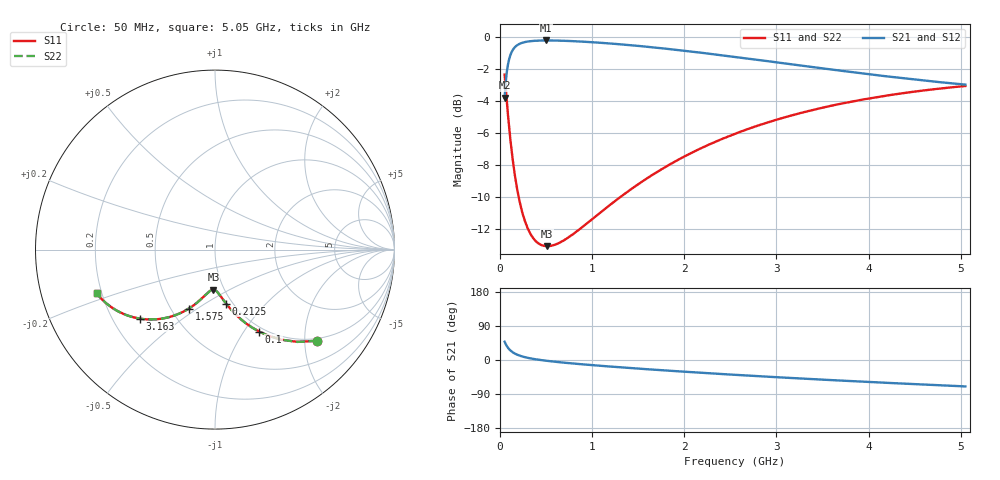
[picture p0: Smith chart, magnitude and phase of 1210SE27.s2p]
! AVX Thin Film Operation		Date: August 2001
! Description: Accu-P® Series, Thin Film, SMD, RF Capacitor
! Part Number: 12101J270FBT
! 50 MHz  -  5.05 GHz
! Serial Measurements
# mhz S db R 50
!	S11		S21		S12		S22
!	dB	Phase	dB	Phase	dB	Phase	dB	Phase
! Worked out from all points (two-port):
!   401 points, 50 MHz to 5.05 GHz, reference 50 ohm
!   highest |S21| = -0.22 dB at 500 MHz (marker M1); lowest = -3.8 dB at 50 MHz (marker M2)
!   |S21| within 3 dB of the highest: 57.29 MHz to end of sweep
!   lowest |S11| = -13.0 dB at 512.5 MHz (marker M3), VSWR 1.57, Z = 44.5 - j20.9 ohm
!   |S11| at or under -10 dB: 203.4 MHz to 1.301 GHz (1.098 GHz wide, 146 % of centre)
!   |S22| runs from -13.0 to -2.3 dB; largest |S21 - S12| = 0
!   S11 on the Smith chart (normalised r, x): 50 MHz: 0.94, -2.29; 100 MHz: 0.94, -1.18; 212.5 MHz: 0.93, -0.62; 1.575 GHz: 0.61, -0.46; 3.163 GHz: 0.31, -0.36; 5.05 GHz: 0.18, -0.17
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50  -2.35 -41.7  -3.80 48.3  -3.80 48.3  -2.35 -41.7
75  -4.10 -53.6  -2.14 36.4  -2.14 36.4  -4.10 -53.6
100  -5.69 -61.6  -1.37 28.3  -1.37 28.3  -5.69 -61.6
125  -7.04 -67.3  -0.96 22.7  -0.96 22.7  -7.04 -67.3
150  -8.17 -71.4  -0.72 18.5  -0.72 18.5  -8.17 -71.5
212.5  -10.25 -78.4  -0.43 11.6  -0.43 11.6  -10.25 -78.4
275  -11.55 -82.8  -0.32 7.2  -0.32 7.2  -11.55 -82.8
337.5  -12.35 -86.0  -0.26 4.0  -0.26 4.0  -12.35 -86.0
412.5  -12.85 -89.0  -0.23 0.9  -0.23 0.9  -12.85 -89.0
500  -13.04 -91.9  -0.22 -1.9  -0.22 -1.9  -13.04 -91.9
512.5  -13.04 -92.2  -0.22 -2.3  -0.22 -2.3  -13.04 -92.2
662.5  -12.78 -96.2  -0.24 -6.3  -0.24 -6.3  -12.78 -96.2
887.5  -11.88 -101.2  -0.29 -11.3  -0.29 -11.3  -11.88 -101.2
1225  -10.34 -107.8  -0.42 -17.8  -0.42 -17.8  -10.34 -107.8
1575  -8.89 -113.9  -0.60 -24.0  -0.60 -24.0  -8.89 -113.9
1725  -8.35 -116.4  -0.69 -26.5  -0.69 -26.5  -8.35 -116.4
2137.5  -7.06 -123.0  -0.96 -33.0  -0.96 -33.0  -7.06 -123.0
2550  -6.04 -129.1  -1.25 -39.1  -1.25 -39.1  -6.04 -129.1
3162.5  -4.90 -137.5  -1.71 -47.5  -1.71 -47.5  -4.90 -137.5
3387.5  -4.56 -140.4  -1.88 -50.4  -1.88 -50.4  -4.56 -140.4
4225  -3.63 -150.5  -2.48 -60.6  -2.48 -60.6  -3.63 -150.5
5050  -3.06 -159.7  -2.98 -69.7  -2.98 -69.7  -3.06 -159.7
